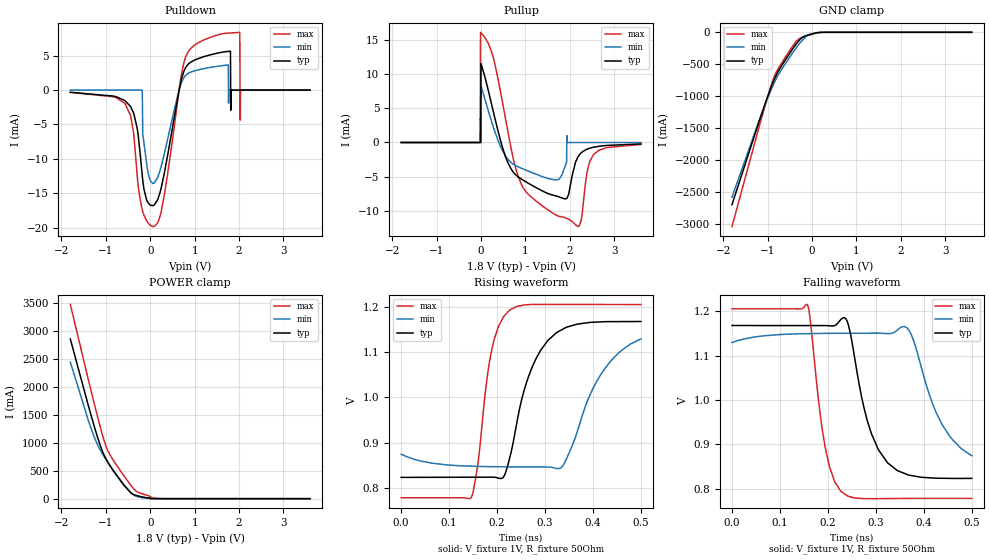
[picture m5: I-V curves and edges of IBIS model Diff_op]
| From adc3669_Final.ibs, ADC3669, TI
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|   Diff_op Model
[Model]   Diff_op
Model_type   Output
Polarity   Non-Inverting
Vmeas = 0.9
Vref = 0.9
Cref = 2pF
Rref = 50
|   typ   min   max
C_comp   0.66pF   0.46pF   0.87pF
| Where C_comp = 0.66pF at 1.8V, 27C and nominal process
| Where C_comp = 0.87pF at 1.75V, 105C and weak process
| Where C_comp = 0.46pF at 2V, -40C and strong process
[Voltage Range]   1.8   1.75   2
|Junction Temperature
[Temperature Range]   27   105   -40
[Pullup Reference]   1.8   1.75   2
[Pulldown Reference]   0   0   -0
[Power Clamp Reference]   1.8   1.75   2
[GND Clamp Reference]   0   0   0
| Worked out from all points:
|   slope of the pulldown table from 0 to 0.27 V, typ, clamps not added: 84.3 ohm
|   slope of the pullup table from 0 to 0.27 V, typ, clamps not added: 39.5 ohm
|   falling waveform, V_fixture 1V, R_fixture 50Ohm: 20-80 % time 48.4ps typ, 56.2ps min, 31.3ps max; typ from 1.17 V to 0.823 V
|   rising waveform, V_fixture 1V, R_fixture 50Ohm: 20-80 % time 56.1ps typ, 68ps min, 30.8ps max; typ from 0.823 V to 1.17 V
[Pulldown]
|   Voltage   I(typ)   I(min)   I(max)
-1.8V     -319.3uA   0A         -320.7uA
-563.4mV  -1.571mA   0A         -2.028mA
-180mV    -12.43mA   0A         -17.38mA
-169.2mV  -13.09mA   -6.445mA   -17.65mA
68.4mV    -16.79mA   -13.57mA   -19.86mA
916.2mV   4.079mA    2.628mA    6.094mA
1.807V    5.662mA    7pA        8.311mA
1.813V    -2.925mA   -15.1pA    8.312mA
2.018V    0A         -41pA      8.412mA
2.023V    0A         -40pA      -4.369mA
2.034V    0A         -40pA      -97.29nA
3.6V      0A         0A         -200pA
[GND Clamp]
|   Voltage   I(typ)   I(min)   I(max)
-1.8V     -2.704A    -2.587A    -3.047A
-1.195V   -1.413A    -1.398A    -1.5A
-1.006V   -1.027A    -1.051A    -1.035A
-887.4mV  -805mA     -853mA     -767.9mA
-790.2mV  -652.5mA   -709.4mA   -610mA
-644.4mV  -483.1mA   -540.6mA   -441.6mA
-444.6mV  -271.4mA   -333.4mA   -225.9mA
-304.2mV  -140.4mA   -199.2mA   -109.5mA
-212.4mV  -79.25mA   -123.2mA   -76.68mA
-109.8mV  -47.36mA   -56.23mA   -54.45mA
171mV     -2.875mA   -2.395mA   -2.761mA
3.6V      0A         0A         0A
[Pullup]
|   Voltage   I(typ)   I(min)   I(max)
-1.8V     0A         0A         0A
-28.8mV   0A         100fA      0A
-18mV     0A         100fA      3.404mA
-12.6mV   0A         100fA      16.15mA
-7.2mV    0A         100fA      16.11mA
-1.8mV    11.55mA    8.256mA    16.07mA
613.8mV   -3.1mA     -2.54mA    1.267mA
1.521V    -7.52mA    -5.295mA   -9.948mA
1.937V    -8.125mA   -90pA      -11.13mA
2.201V    -1.92mA    0A         -12.27mA
2.525V    -704.3uA   0A         -1.844mA
3.6V      -214.6uA   0A         -288.9uA
[POWER Clamp]
|   Voltage   I(typ)   I(min)   I(max)
-1.8V     2.851A     2.439A     3.468A
-1.406V   1.695A     1.428A     2.164A
-1.287V   1.362A     1.155A     1.78A
-1.114V   922.8mA    851.5mA    1.246A
-1.006V   724.1mA    710.4mA    958.5mA
-865.8mV  538.6mA    541mA      727.3mA
-595.8mV  242.9mA    254.7mA    411.5mA
-444.6mV  109mA      116.8mA    246.3mA
-331.2mV  61.6mA     48.17mA    144.1mA
-12.6mV   11.12mA    6.394mA    33.58mA
235.8mV   23.88uA    6.093uA    1.737mA
3.6V      0A         0A         0A
[Ramp]
R_load = 50
|   typ   min   max
dV/dt_r   0.206665/5.60632e-11   0.152923/6.80201e-11   0.256207/3.08482e-11
dV/dt_f   0.206655/4.84618e-11   0.152923/5.61731e-11   0.256204/3.13463e-11
[Falling Waveform]
V_fixture = 1V
V_fixture_min = 1V
V_fixture_max = 1V
R_fixture = 50Ohm
C_fixture = 0F
|   Time   V(typ)   V(min)   V(max)
0s        1.168V     1.13V      1.205V
156.5ps   1.168V     1.149V     1.215V
193.8ps   1.168V     1.15V      896.5mV
214.2ps   1.168V     1.15V      815.8mV
237.1ps   1.184V     1.15V      786.7mV
290.8ps   924.2mV    1.151V     777.8mV
324.3ps   858.7mV    1.15V      778mV
360.7ps   834.2mV    1.165V     778.3mV
437.3ps   823.7mV    946.2mV    778.4mV
500ps     823.5mV    874.6mV    778.4mV
[Rising Waveform]
V_fixture = 1V
V_fixture_min = 1V
V_fixture_max = 1V
R_fixture = 50Ohm
C_fixture = 0F
|   Time   V(typ)   V(min)   V(max)
0s        823.4mV    874.6mV    778.3mV
146.7ps   823.7mV    848.2mV    779.8mV
160.6ps   823.8mV    847.7mV    857.6mV
188ps     823.8mV    847.1mV    1.101V
226.8ps   868mV      846.6mV    1.193V
261.2ps   1.032V     846.5mV    1.205V
305.5ps   1.126V     846.3mV    1.206V
338.1ps   1.151V     850.1mV    1.206V
425.7ps   1.167V     1.065V     1.205V
500ps     1.168V     1.13V      1.205V
